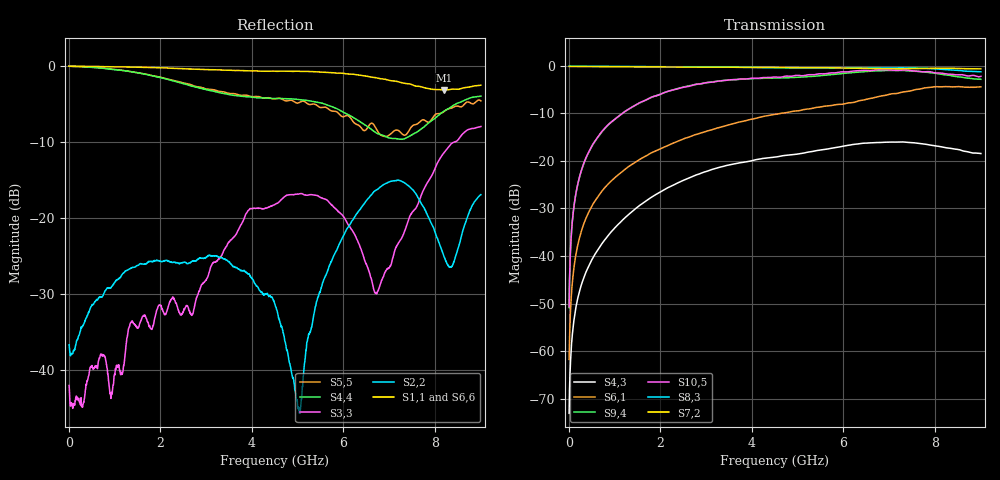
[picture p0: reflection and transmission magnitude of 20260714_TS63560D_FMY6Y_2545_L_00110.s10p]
# GHz S DB R 50
! CMT, SN0916, 25263762, 26.7.0
! Date: 15.07.2026 13:35:54
! Data: Format
! Freq S1.1:dB/Ang S1.2:dB/Ang S1.3:dB/Ang S1.4:dB/Ang S1.5:dB/Ang S1.6:dB/Ang S1.7:dB/Ang S1.8:dB/Ang S1.9:dB/Ang S1.10:dB/Ang
!  S2.1:dB/Ang S2.2:dB/Ang S2.3:dB/Ang S2.4:dB/Ang S2.5:dB/Ang S2.6:dB/Ang S2.7:dB/Ang S2.8:dB/Ang S2.9:dB/Ang S2.10:dB/Ang
!  S3.1:dB/Ang S3.2:dB/Ang S3.3:dB/Ang S3.4:dB/Ang S3.5:dB/Ang S3.6:dB/Ang S3.7:dB/Ang S3.8:dB/Ang S3.9:dB/Ang S3.10:dB/Ang
!  S4.1:dB/Ang S4.2:dB/Ang S4.3:dB/Ang S4.4:dB/Ang S4.5:dB/Ang S4.6:dB/Ang S4.7:dB/Ang S4.8:dB/Ang S4.9:dB/Ang S4.10:dB/Ang
!  S5.1:dB/Ang S5.2:dB/Ang S5.3:dB/Ang S5.4:dB/Ang S5.5:dB/Ang S5.6:dB/Ang S5.7:dB/Ang S5.8:dB/Ang S5.9:dB/Ang S5.10:dB/Ang
!  S6.1:dB/Ang S6.2:dB/Ang S6.3:dB/Ang S6.4:dB/Ang S6.5:dB/Ang S6.6:dB/Ang S6.7:dB/Ang S6.8:dB/Ang S6.9:dB/Ang S6.10:dB/Ang
!  S7.1:dB/Ang S7.2:dB/Ang S7.3:dB/Ang S7.4:dB/Ang S7.5:dB/Ang S7.6:dB/Ang S7.7:dB/Ang S7.8:dB/Ang S7.9:dB/Ang S7.10:dB/Ang
!  S8.1:dB/Ang S8.2:dB/Ang S8.3:dB/Ang S8.4:dB/Ang S8.5:dB/Ang S8.6:dB/Ang S8.7:dB/Ang S8.8:dB/Ang S8.9:dB/Ang S8.10:dB/Ang
!  S9.1:dB/Ang S9.2:dB/Ang S9.3:dB/Ang S9.4:dB/Ang S9.5:dB/Ang S9.6:dB/Ang S9.7:dB/Ang S9.8:dB/Ang S9.9:dB/Ang S9.10:dB/Ang
!  S10.1:dB/Ang S10.2:dB/Ang S10.3:dB/Ang S10.4:dB/Ang S10.5:dB/Ang S10.6:dB/Ang S10.7:dB/Ang S10.8:dB/Ang S10.9:dB/Ang S10.10:dB/Ang
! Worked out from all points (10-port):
!   2001 points, 10 MHz to 9 GHz, reference 50 ohm
!   strongest paths, dB at 10 MHz, 2.257 GHz, 4.505 GHz, 6.753 GHz, 9 GHz:
!     S7,2: -0.1, -0.2, -0.3, -0.6, -0.6
!     S8,3: -0.1, -0.2, -0.4, -0.4, -1.3
!     S10,5: -50.7, -5.1, -2.3, -0.8, -2.2
!     S9,4: -50.8, -5.1, -2.6, -1.0, -2.8
!     S6,1: -61.7, -16.4, -10.2, -6.5, -4.4
!     S4,3: -73.1, -25.2, -19.2, -16.1, -18.4
!   lowest |S11| = -3.1 dB at 8.2 GHz (marker M1), VSWR 5.61, Z = 11.1 - j24 ohm
!   |S11| at or under -10 dB: nowhere
